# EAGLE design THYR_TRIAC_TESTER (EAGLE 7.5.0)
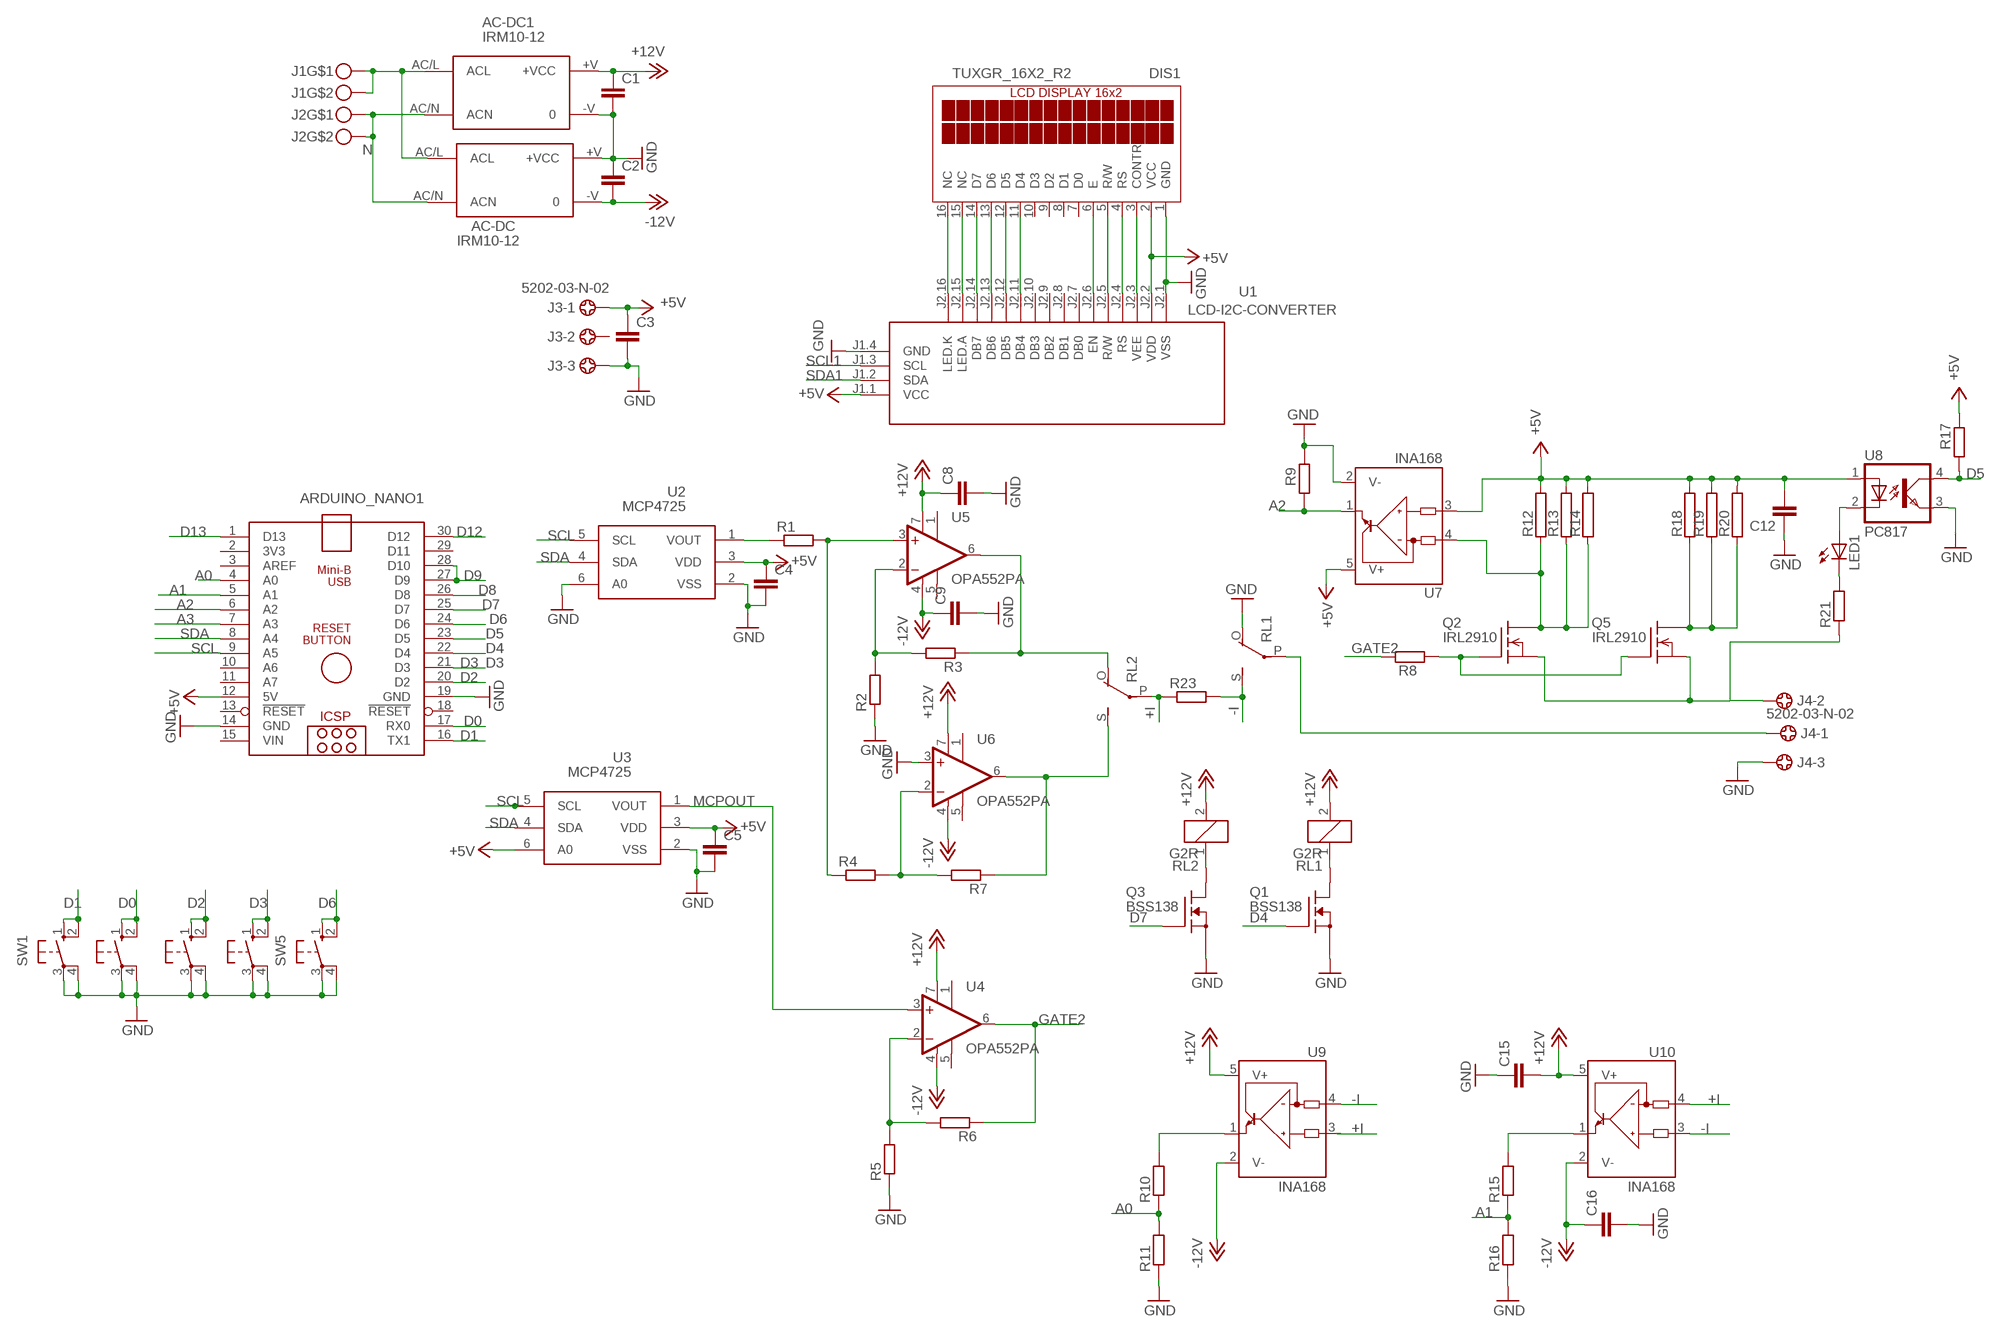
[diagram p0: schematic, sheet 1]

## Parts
AC-DC  IRM10-12  [IRM10-12]
AC-DC1  IRM10-12  [IRM10-12]
ARDUINO_NANO1  ARDUINO_NANO  [ARDUINO_NANO]
C1  C-EUC1206  [C1206]
C2  C-EUC1206  [C1206]
C3  C-EUC1206  [C1206]
C4  C-EUC1206  [C1206]
C5  C-EUC1206  [C1206]
C8  C-EUC1206  [C1206]
C9  C-EUC1206  [C1206]
C12  C-EUC1206  [C1206]
C15  C-EUC1206  [C1206]
C16  C-EUC1206  [C1206]
DIS1  TUXGR_16X2_R2  [TUXGR_16X2_R2]
J1  MKDSN1,5-2-5,08  [MKDSN1,5-2-5,08]
J2  MKDSN1,5-2-5,08  [MKDSN1,5-2-5,08]
J3  5202-03-N-02  [5202-03-N-02]
J4  5202-03-N-02  [5202-03-N-02]
LED1  LED5MM  [LED5MM]
Q1  BSS138  [SOT23]
Q2  IRL2910  SUP75N06-08  [TO220]
Q3  BSS138  [SOT23]
Q5  IRL2910  SUP75N06-08  [TO220]
R1  R-EU_M1206  [M1206]
R2  R-EU_M1206  [M1206]
R3  R-EU_M1206  [M1206]
R4  R-EU_M1206  [M1206]
R5  R-EU_M1206  [M1206]
R6  R-EU_M1206  [M1206]
R7  R-EU_M1206  [M1206]
R8  R-EU_M1206  [M1206]
R9  R-EU_M1206  [M1206]
R10  R-EU_M1206  [M1206]
R11  R-EU_M1206  [M1206]
R12  RRWM10X65  [RWM10X65]
R13  RRWM10X65  [RWM10X65]
R14  RRWM10X65  [RWM10X65]
R15  R-EU_M1206  [M1206]
R16  R-EU_M1206  [M1206]
R17  R-EU_M1206  [M1206]
R18  RRWM10X65  [RWM10X65]
R19  RRWM10X65  [RWM10X65]
R20  RRWM10X65  [RWM10X65]
R21  R-EU_M1206  [M1206]
R23  R-EU_R2512  [R2512]
RL1  G2R  [G2R]
RL2  G2R  [G2R]
SW1  40-XX  [B3F-40XX]
SW2  40-XX  [B3F-40XX]
SW3  40-XX  [B3F-40XX]
SW4  40-XX  [B3F-40XX]
SW5  40-XX  [B3F-40XX]
U1  LCD-I2C-CONVERTER  [LCD-I2C-CONVERTER]
U2  MCP4725  [SOT23-6]
U3  MCP4725  [SOT23-6]
U4  OPA552PA  OPA627U  [SO08]
U5  OPA552PA  OPA627U  [SO08]
U6  OPA552PA  OPA627U  [SO08]
U7  INA168  [SOT23-5]
U8  PC817  [DIL04]
U9  INA168  [SOT23-5]
U10  INA168  [SOT23-5]

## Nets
+5V: ARDUINO_NANO1.12(5V) C3.1 C4.1 C5.1 C12.2 DIS1.2(VCC) J3.1 R12.2 R13.2 R14.2 R17.2 R18.2 R19.2 R20.2 U1.J1.1(VCC) U1.J2.2(VDD) U2.3(VDD) U3.3(VDD) U3.6(A0) U7.3(IN+) U7.5(V+) U8.1(A)
+12V: AC-DC1.+V(+VCC) C1.1 C8.1 C15.2 RL1.2 RL2.2 U4.7(V+) U5.7(V+) U6.7(V+) U9.5(V+) U10.5(V+)
+I: R23.1 RL2.P(2:P) U10.4(IN-)
-12V: AC-DC.-V C2.2 C9.1 C16.1 U4.4(V-) U5.4(V-) U6.4(V-) U9.2(V-) U10.2(V-)
-I: R23.2 RL1.S(2:S) U9.4(IN-) U10.3(IN+)
A0: ARDUINO_NANO1.4(A0) R10.1 R11.2
A1: ARDUINO_NANO1.5(A1) R15.1 R16.2
A2: ARDUINO_NANO1.6(A2) R9.1 U7.1(OUT)
A3: ARDUINO_NANO1.7(A3)
D0: ARDUINO_NANO1.17(RX0) SW2.1(S) SW2.2(S1)
D1: ARDUINO_NANO1.16(TX1) SW1.1(S) SW1.2(S1)
D2: ARDUINO_NANO1.20(D2) SW3.1(S) SW3.2(S1)
D3: ARDUINO_NANO1.21(D3) SW4.1(S) SW4.2(S1)
D4: ARDUINO_NANO1.22(D4) Q1.3(G)
D5: ARDUINO_NANO1.23(D5) R17.1 U8.4(COL)
D6: ARDUINO_NANO1.24(D6) SW5.1(S) SW5.2(S1)
D7: ARDUINO_NANO1.25(D7) Q3.3(G)
D8: ARDUINO_NANO1.26(D8)
D9: ARDUINO_NANO1.27(D9) ARDUINO_NANO1.28(D10)
D12: ARDUINO_NANO1.30(D12)
D13: ARDUINO_NANO1.1(D13)
GATE2: R6.1 R8.2 U4.6(OUT)
GND: AC-DC1.-V AC-DC.+V(+VCC) ARDUINO_NANO1.14(GND) ARDUINO_NANO1.19(GND) C1.2 C2.1 C3.2 C4.2 C5.2 C8.2 C9.2 C12.1 C15.1 C16.2 DIS1.1(GND) J3.3 J4.3 Q1.1(S) Q3.1(S) R2.1 R5.1 R9.2 R11.1 R16.1 RL1.O(2:O) SW1.3(P) SW1.4(P1) SW2.3(P) SW2.4(P1) SW3.3(P) SW3.4(P1) SW4.3(P) SW4.4(P1) SW5.3(P) SW5.4(P1) U1.J1.4(GND) U1.J2.1(VSS) U2.2(VSS) U2.6(A0) U3.2(VSS) U6.3(+IN) U7.2(V-) U8.3(EMIT)
MCPOUT: U3.1(VOUT) U4.3(+IN)
N: AC-DC1.AC/N(ACN) AC-DC.AC/N(ACN) J2.1 J2.2
N$1: R1.1 U2.1(VOUT)
N$2: R1.2 R4.1 U5.3(+IN)
N$3: R3.1 RL2.O(2:O) U5.6(OUT)
N$4: AC-DC1.AC/L(ACL) AC-DC.AC/L(ACL) J1.1 J1.2
N$5: R2.2 R3.2 U5.2(-IN)
N$6: Q3.2(D) RL2.1
N$7: R7.1 RL2.S(2:S) U6.6(OUT)
N$8: R4.2 R7.2 U6.2(-IN)
N$9: Q2.1(G) Q5.1(G) R8.1
N$10: R5.2 R6.2 U4.2(-IN)
N$11: R10.2 U9.1(OUT)
N$12: Q1.2(D) RL1.1
N$13: LED1.A U8.2(C)
N$14: Q2.2(D) R12.1 R13.1 R14.1 U7.4(IN-)
N$15: Q5.2(D) R18.1 R19.1 R20.1
N$16: LED1.K(C) R21.2
N$18: R15.2 U10.1(OUT)
N$19: J4.1 RL1.P(2:P)
N$20: J4.2 Q2.3(S) Q5.3(S) R21.1
N$31: DIS1.3(CONTR) U1.J2.3(VEE)
N$32: DIS1.4(RS) U1.J2.4(RS)
N$33: DIS1.5(R/W) U1.J2.5(R/W)
N$34: DIS1.6(E) U1.J2.6(EN)
N$35: DIS1.14(D7) U1.J2.14(DB7)
N$36: DIS1.13(D6) U1.J2.13(DB6)
N$37: DIS1.12(D5) U1.J2.12(DB5)
N$38: DIS1.11(D4) U1.J2.11(DB4)
N$39: DIS1.16(NC) U1.J2.16(LED.K)
N$40: DIS1.15(NC) U1.J2.15(LED.A)
SCL: ARDUINO_NANO1.9(A5) U2.5(SCL) U3.5(SCL)
SCL1: U1.J1.3(SCL)
SDA: ARDUINO_NANO1.8(A4) U2.4(SDA) U3.4(SDA)
SDA1: U1.J1.2(SDA)
Unconnected: ARDUINO_NANO1.2(3V3) ARDUINO_NANO1.3(AREF) ARDUINO_NANO1.10(A6) ARDUINO_NANO1.11(A7) ARDUINO_NANO1.13(!RESET) ARDUINO_NANO1.18(!RESET) ARDUINO_NANO1.29(D11) DIS1.7(D0) DIS1.8(D1) DIS1.9(D2) DIS1.10(D3) J3.2 U1.J2.7(DB0) U1.J2.8(DB1) U1.J2.9(DB2) U1.J2.10(DB3) U4.1(TRIM1) U4.5(TRIM2) U5.1(TRIM1) U5.5(TRIM2) U6.1(TRIM1) U6.5(TRIM2) U9.3(IN+)

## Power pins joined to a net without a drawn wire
VIN: ARDUINO_NANO1.15(VIN)

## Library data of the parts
AC-DC AC-DC1 = acdc:IRM10-12
ARDUINO_NANO1 = ArduinoNanoV30:ARDUINO_NANO: Arduino Nano V3.0 Overview: The Arduino Nano is a small, complete, and breadboard-friendly board based on the ATmega328 (Arduino Nano 3.x) or ATmega168 (Arduino Nano 2.x). It has more or less the same functionality of the Arduino Duemilanove, but in a different package. It lacks only a DC power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
C1-C5 C8 C9 C12 C15 C16 = rcl:C-EU: CAPACITOR, European symbol
DIS1 = display-lcd:TUXGR_16X2_R2: Tuxgraphics LCD display 16x2 characters reflective, without background light Source: tuxgr_12x2_r2.pdf; OC_FARNELL: unknown; OC_NEWARK: unknown
J1 J2 = con-phoenix-508:MKDSN1,5-2-5,08
J3 J4 = con-ebyelectro:5202-03-N-02: Barrier Blocks Sreies 5202 Source: http://www.ebyelectro.com/PDF/5202-XX-N-02.pdf; OC_FARNELL: unknown; OC_NEWARK: unknown
LED1 = led:LED: LED
Q1 Q3 = transistor-fet:BSS138
Q2 Q5 = transistor-fet:SUP75N06-08: N-Channel Enhancement MOSFET 60V; 75A; 0,008Ohm
R1-R11 R15-R17 R21 R23 = rcl:R-EU_: RESISTOR, European symbol
R12-R14 R18-R20 = resistor-power:R: Power Resitor; OC_FARNELL: unknown; OC_NEWARK: unknown
RL1 RL2 = relay:G2R: RELAY 1 x switch, Omron; OC_FARNELL: 1569185; OC_NEWARK: unknown
SW1-SW5 = switch-omron:40-XX: OMRON SWITCH; MF: OMRON COMPONENTS USA; MPN: B3F-4000; OC_FARNELL: 176434; OC_NEWARK: 36K3105
U1 = diy-modules:LCD-I2C-CONVERTER: I2C Bus to 4-Bit Parallel LCD Interface with LED backlight driver
U2 U3 = linear:MCP4725
U4-U6 = burr-brown:OPA627: Difet(R) Operational Amplifiers Precision, High-Speed; MF: TEXAS INSTRUMENTS; MPN: OPA627AU; OC_FARNELL: 1207067; OC_NEWARK: 30C4516
U7 U9 U10 = burr-brown:INA168: High-Side Measurement Current Shunt Monitor; MF: TEXAS INSTRUMENTS; MPN: INA168NA/250; OC_FARNELL: 4375737; OC_NEWARK: 35C1744
U8 = optocoupler:PC817: SHARP OPTO COUPLER; MPN: PC817X4J000F; OC_FARNELL: 9707727; OC_NEWARK: 97K7059

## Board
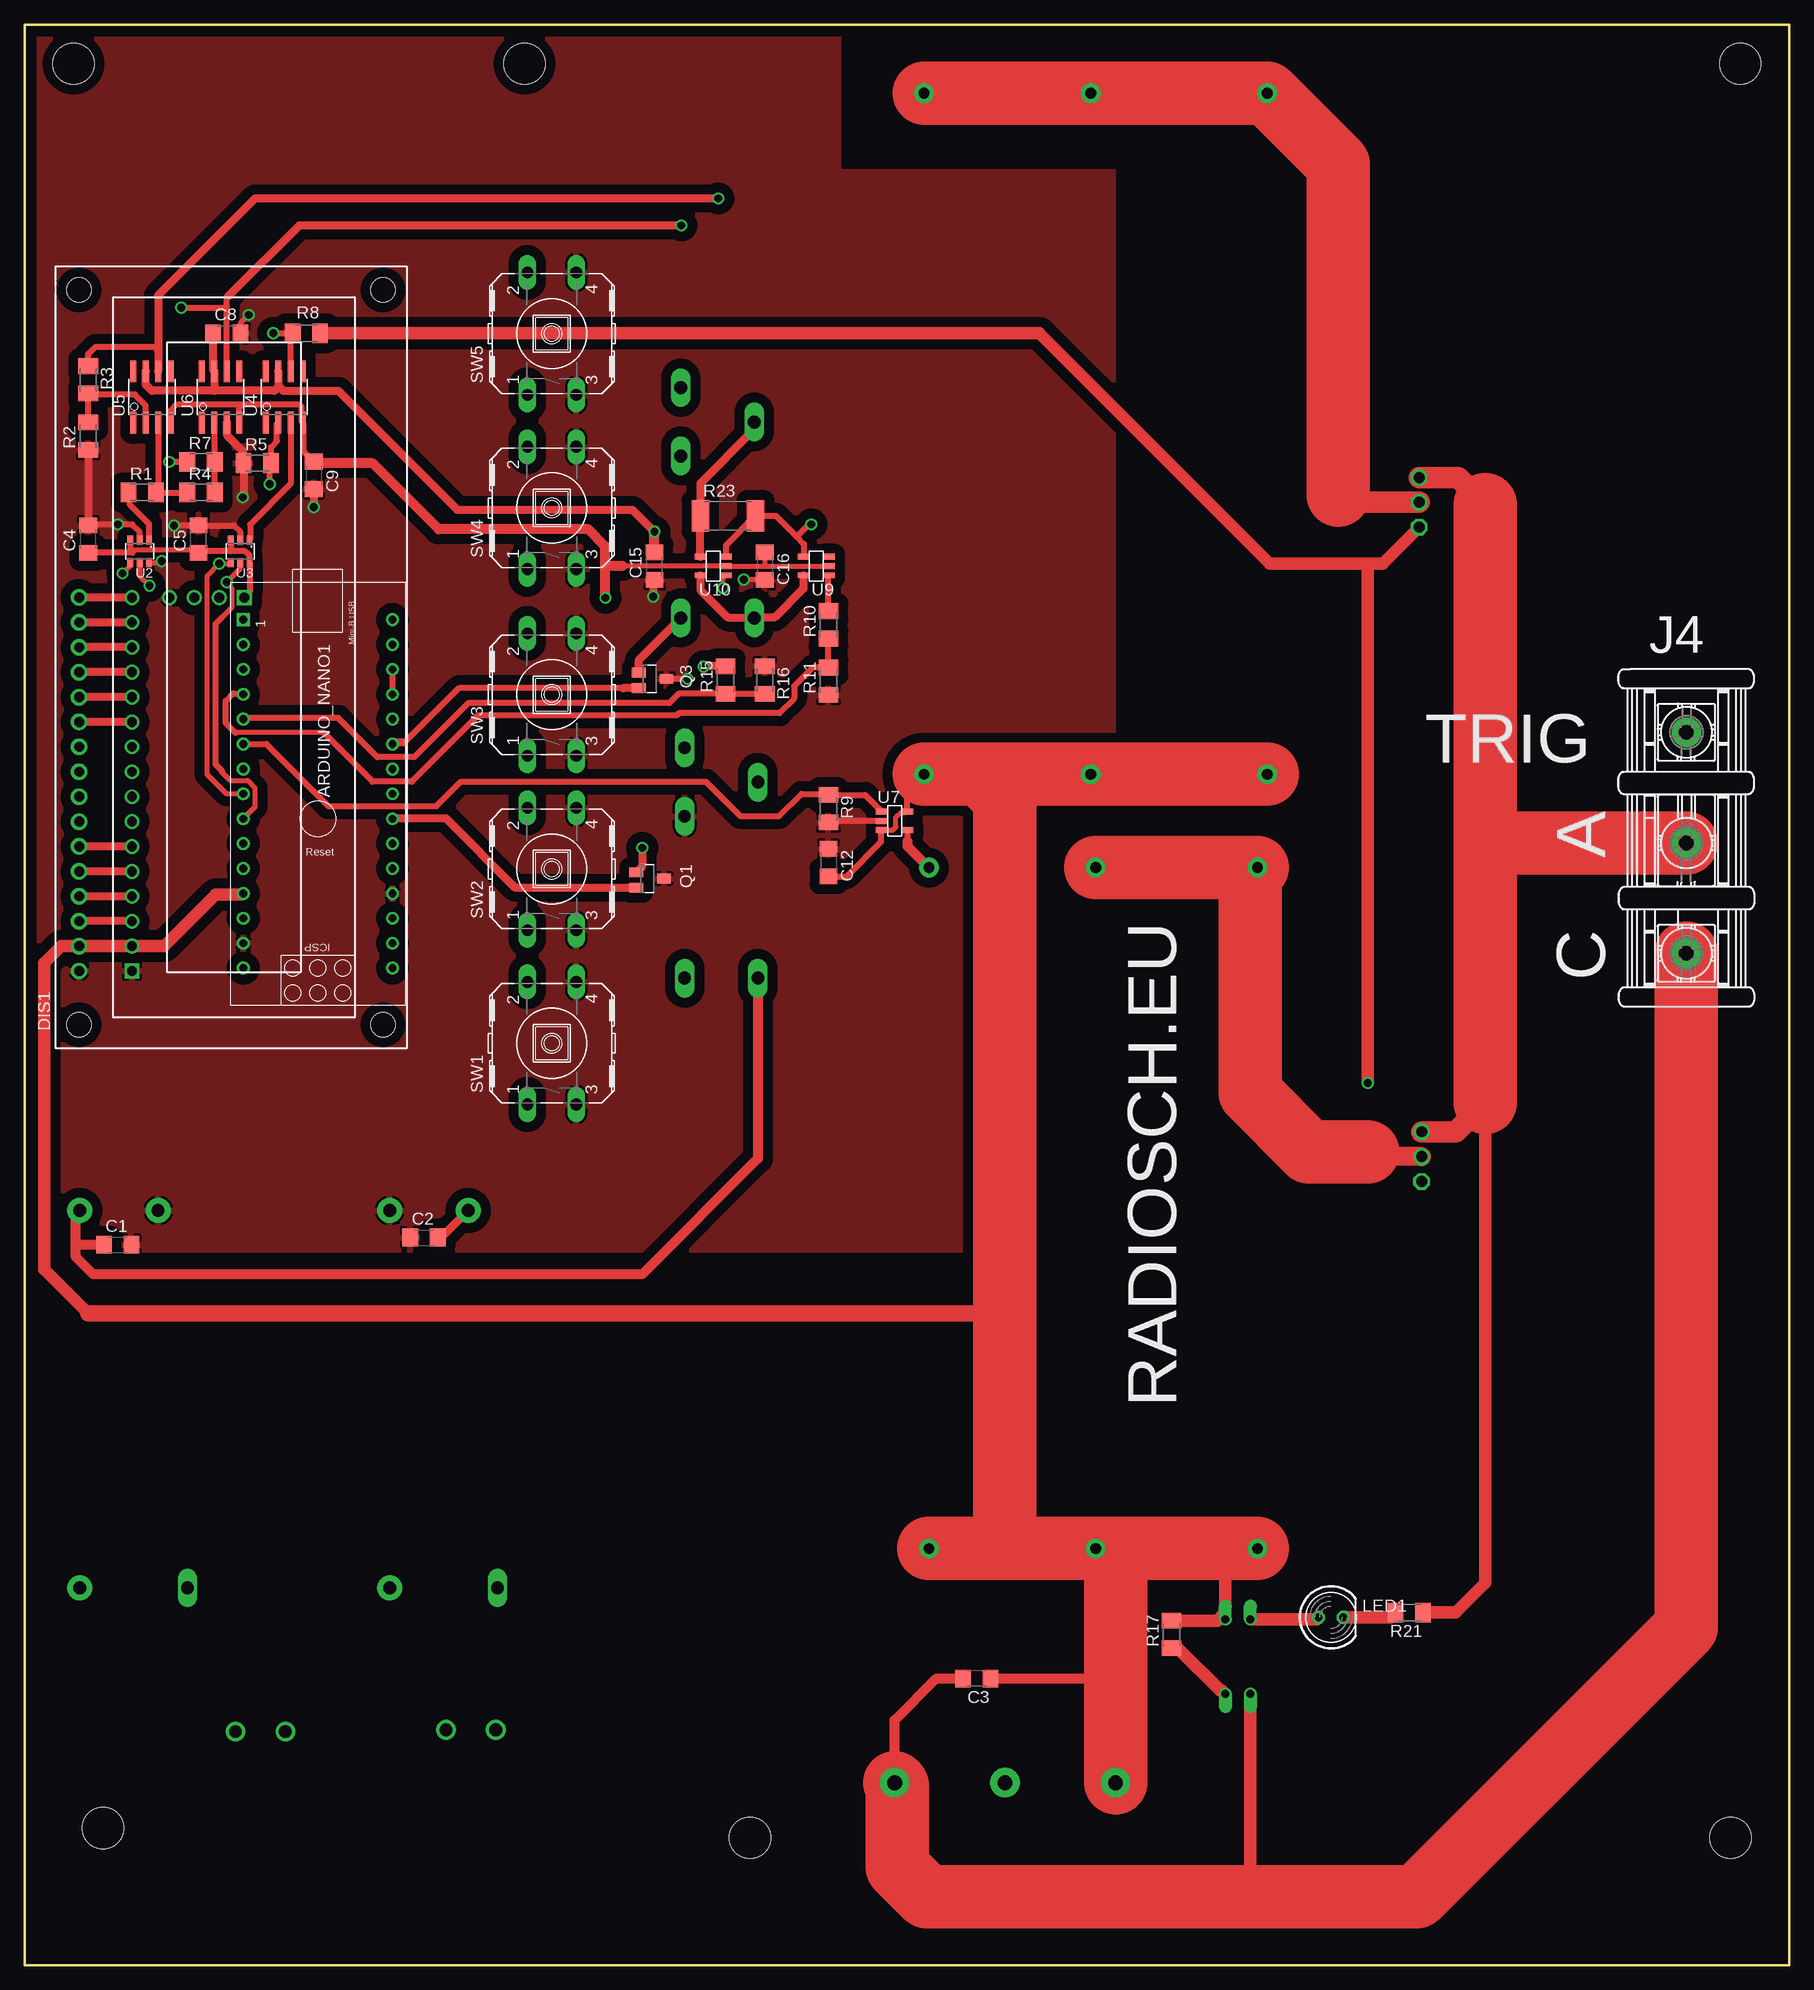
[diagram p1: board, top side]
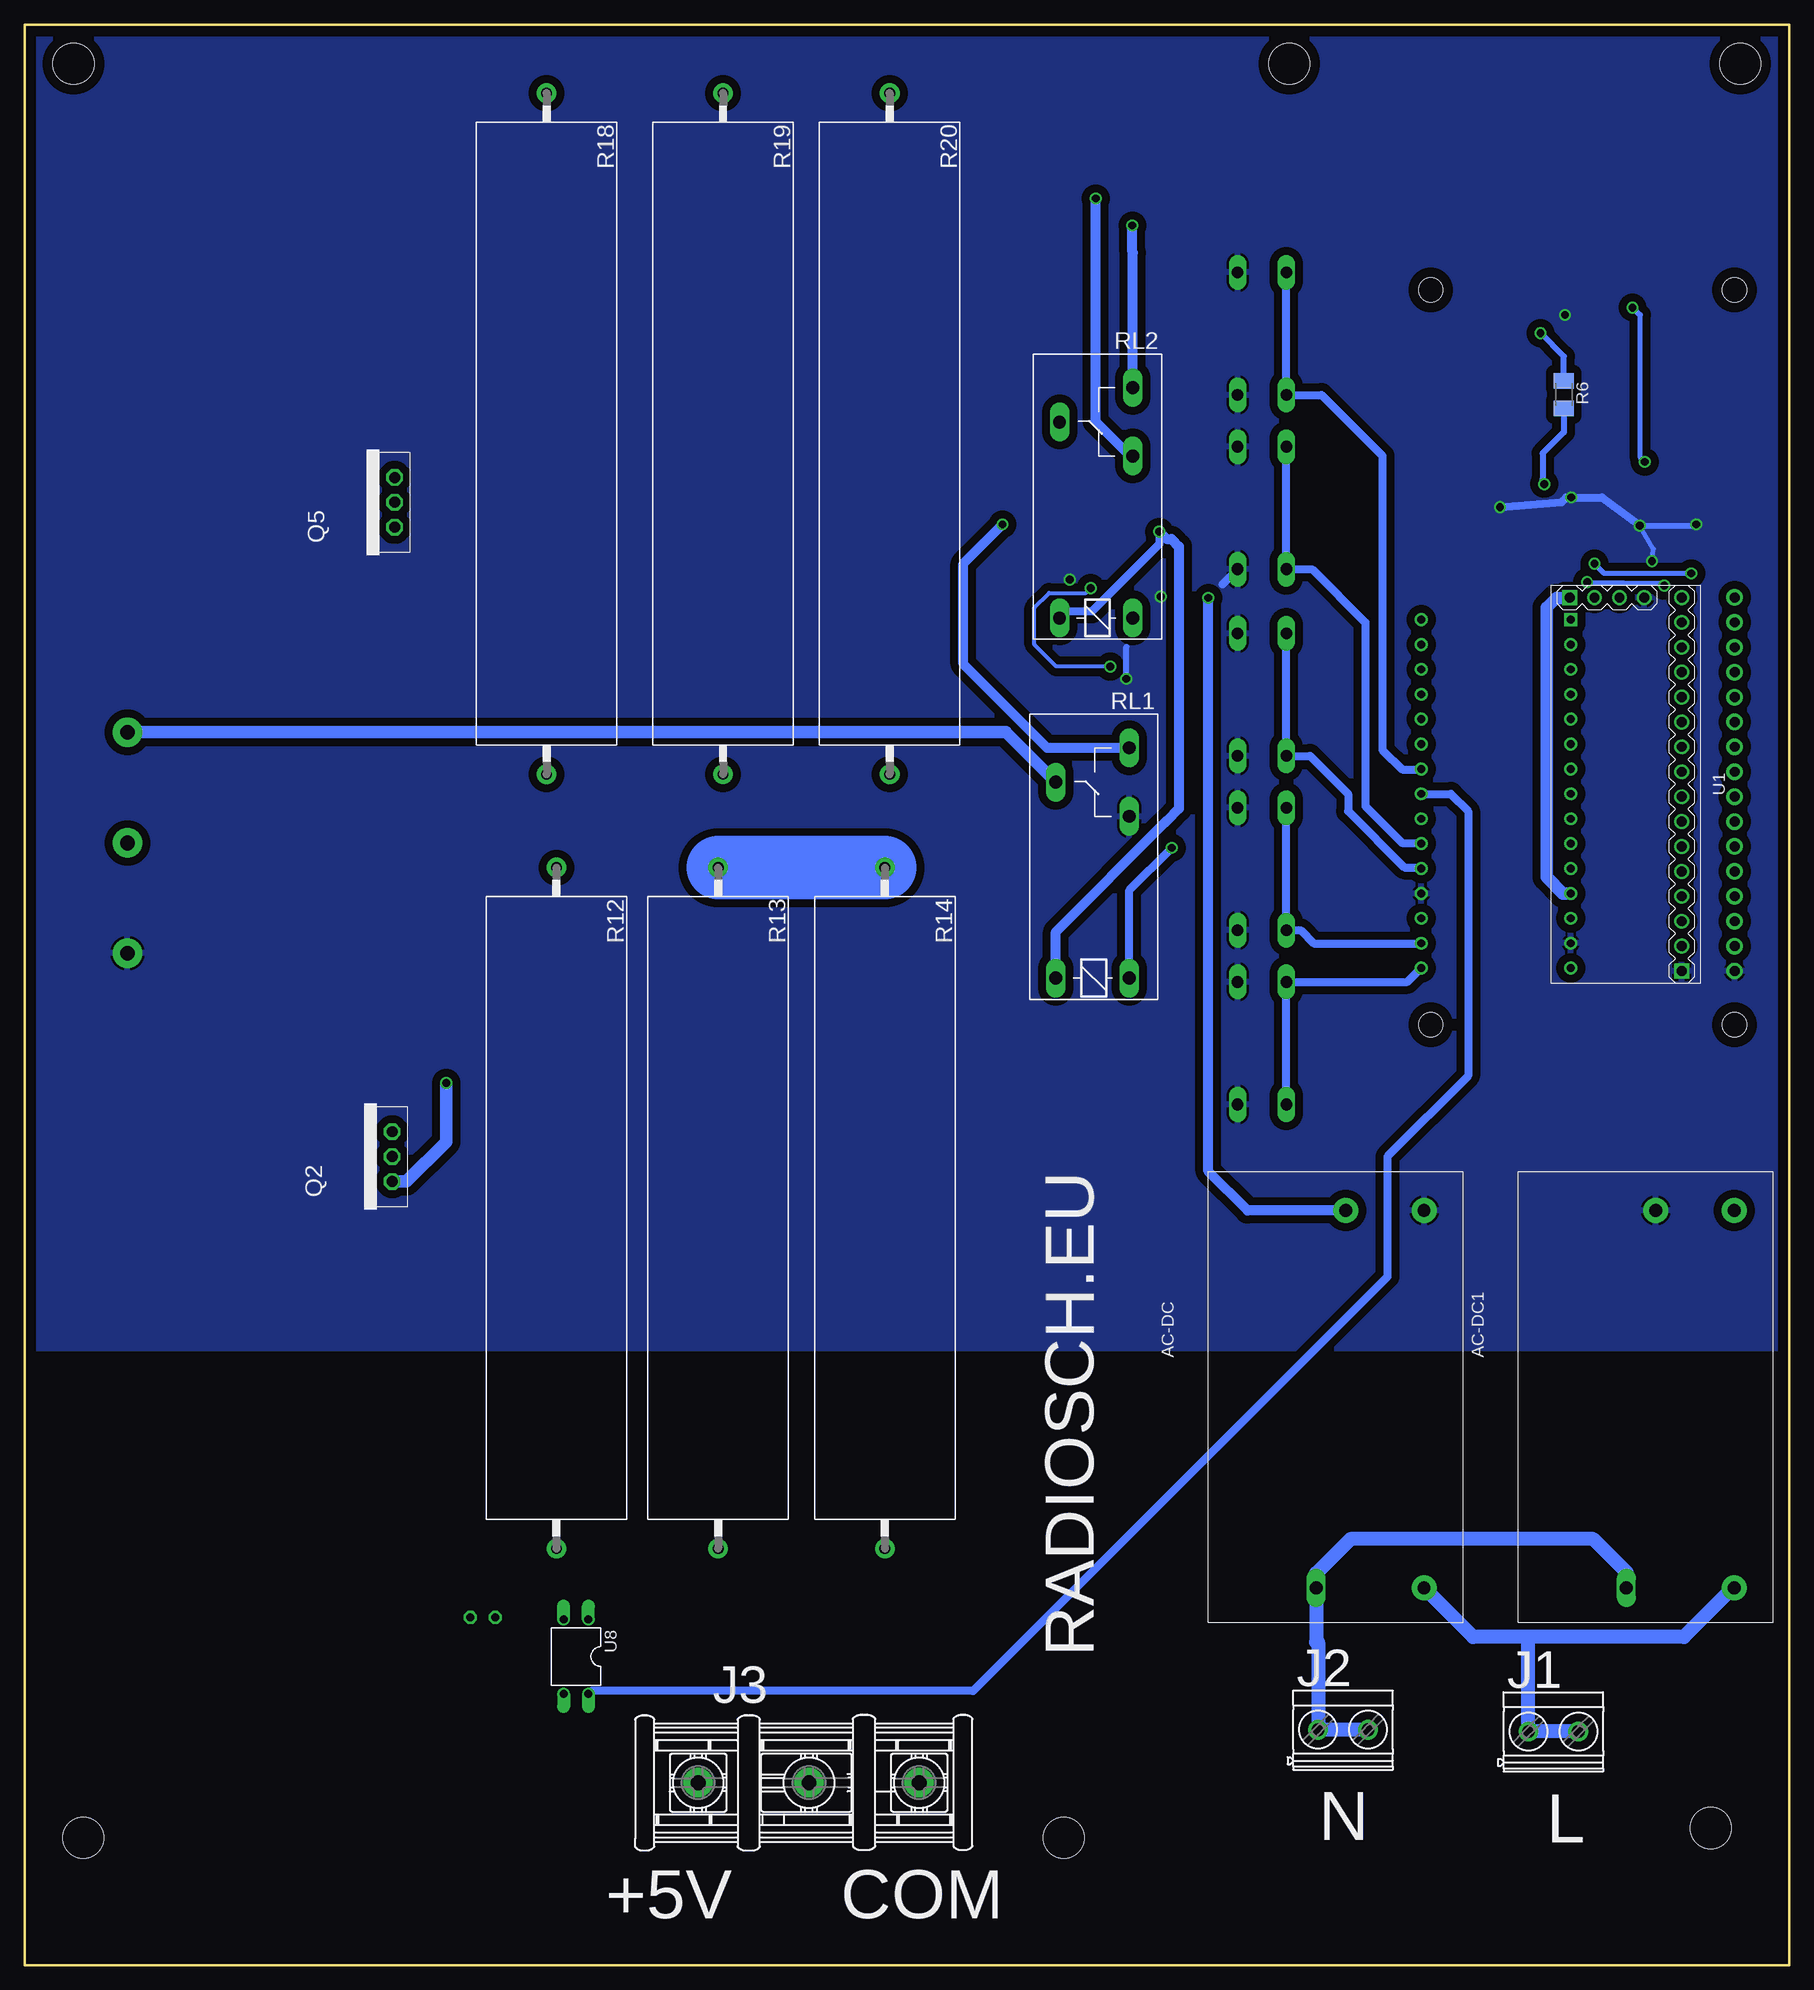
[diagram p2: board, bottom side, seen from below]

Size 180 x 198 mm. Coordinates in mm from the lower left corner, seen from the top.
Outline: 0,0 180,0 180,198 0,198 0,0
Copper layers (1*16): Top 0.035mm / dielectric 1.5mm / Bottom 0.035mm
Design rules "default": minimum track width 10mil, minimum drill 24mil, track to track 8mil, track to pad 8mil, pad to pad 8mil, via to via 8mil, smd to smd 8mil, copper to edge 40mil, drill to drill 8mil, minimum pad ring 10mil, minimum via ring 8mil, stop-mask expansion 4mil, vias tented up to drill 0mil, thermal gap 10mil
Holes 4.2 mm at 5,194 51,194 175,194 8,14 74,13 174,13

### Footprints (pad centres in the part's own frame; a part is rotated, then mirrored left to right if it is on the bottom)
IRM10-12 = drill 1.3 pad 2.54: +V 38.5,0; -V 38.5,8; AC/L 0,0 | drill 1.3 long: AC/N 0,11
ARDUINO_NANO = drill 0.8 square: 1 -20.32,-7.62 | drill 0.8: 2 -17.78,-7.62; 3 -15.24,-7.62; 4 -12.7,-7.62; 5 -10.16,-7.62; 6 -7.62,-7.62; 7 -5.08,-7.62; 8 -2.54,-7.62; 9 0,-7.62; 10 2.54,-7.62; 11 5.08,-7.62; 12 7.62,-7.62; 13 10.16,-7.62; 14 12.7,-7.62; 15 15.24,-7.62; 16 15.24,7.62; 17 12.7,7.62; 18 10.16,7.62; 19 7.62,7.62; 20 5.08,7.62; 21 2.54,7.62; 22 0,7.62; 23 -2.54,7.62; 24 -5.08,7.62; 25 -7.62,7.62; 26 -10.16,7.62; 27 -12.7,7.62; 28 -15.24,7.62; 29 -17.78,7.62; 30 -20.32,7.62
C1206 = smd 1.6 x 1.8: 1 -1.4,0; 2 1.4,0
TUXGR_16X2_R2 = drill 1 pad 1.676: 1 -32,15.5; 2 -29.46,15.5; 3 -26.92,15.5; 4 -24.38,15.5; 5 -21.84,15.5; 6 -19.3,15.5; 7 -16.76,15.5; 8 -14.22,15.5; 9 -11.68,15.5; 10 -9.14,15.5; 11 -6.6,15.5; 12 -4.06,15.5; 13 -1.52,15.5; 14 1.02,15.5; 15 3.56,15.5; 16 6.1,15.5 | hole 2.5: -37.5,-15.5; 37.5,-15.5; -37.5,15.5; 37.5,15.5
MKDSN1,5-2-5,08 = drill 1.3 pad 2: 1 -2.561,0.025; 2 2.519,0.025
5202-03-N-02 = drill 1.5 pad 3: 1 -9.29,0; 2 2,0; 3 13.25,0
LED5MM = drill 0.813 octagon: A -1.27,0; K 1.27,0
SOT23 = smd 1 x 1.4: 1 0,1.735; 2 -0.632,-1.1; 3 0.95,-1.1
TO220 = drill 1.118 octagon: 1 -2.54,0; 2 0,0; 3 2.54,0
M1206 = smd 1.6 x 2: 1 -1.4,0; 2 1.4,0
RWM10X65 = drill 1.1 pad 2: 1 -34.74,0; 2 34.74,0
R2512 = smd 1.8 x 3.2: 1 -2.8,0; 2 2.8,0
G2R = drill 1.321 long: 1 -2.54,-3.683; 2 -2.54,3.81; O 13.97,-3.683; P 17.45,3.81; S 20.955,-3.683
B3F-40XX = drill 1.194 long: 1 -6.248,2.489; 2 6.248,2.489; 3 -6.248,-2.489; 4 6.248,-2.489
LCD-I2C-CONVERTER = drill 1 square: J1.1 -19.05,-5.08; J2.1 19.05,6.35 | drill 1: J1.2 -19.05,-2.54; J1.3 -19.05,0; J1.4 -19.05,2.54; J2.2 16.51,6.35; J2.3 13.97,6.35; J2.4 11.43,6.35; J2.5 8.89,6.35; J2.6 6.35,6.35; J2.7 3.81,6.35; J2.8 1.27,6.35; J2.9 -1.27,6.35; J2.10 -3.81,6.35; J2.11 -6.35,6.35; J2.12 -8.89,6.35; J2.13 -11.43,6.35; J2.14 -13.97,6.35; J2.15 -16.51,6.35; J2.16 -19.05,6.35
SOT23-6 = smd 0.6 x 0.9: 1 -0.95,-1.15; 2 0,-1.15; 3 0.95,-1.15; 4 0.95,1.15; 5 0,1.15; 6 -0.95,1.15
SO08 = smd 0.61 x 2.21: 1 -1.905,-2.616; 2 -0.635,-2.616; 3 0.635,-2.616; 4 1.905,-2.616; 5 1.905,2.616; 6 0.635,2.616; 7 -0.635,2.616; 8 -1.905,2.616
SOT23-5 = smd 0.6 x 1.2: 1 -0.95,-1.306; 2 0,-1.306; 3 0.95,-1.306; 4 0.95,1.306; 5 -0.95,1.306
DIL04 = drill 0.813 offset: 1 -1.27,-3.81; 2 1.27,-3.81; 3 1.27,3.81; 4 -1.27,3.81

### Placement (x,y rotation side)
AC-DC  37.25,38.5 90 bottom
AC-DC1  5.62,38.5 90 bottom
ARDUINO_NANO1  29.92,116.97 270 top
C1  9.5,73.5 0 top
C2  40.75,74.25 0 top
C3  97.12,29.25 180 top
C4  6.5,145.5 90 top
C5  17.75,145.5 90 top
C8  20.62,166.5 0 top
C9  29.5,152 270 top
C12  82,112.5 270 top
C15  64.25,142.75 90 top
C16  75.5,142.75 270 top
DIS1  21.07,133.44 90 top
J1  24.04,23.82 0 bottom
J2  45.5,24 0 bottom
J3  102,18.62 0 bottom
J4  169.5,116.5 270 top
LED1  133.25,35.5 0 top
Q1  63.5,110.88 270 top
Q2  142.5,82.5 90 bottom
Q3  63.75,131.25 270 top
Q5  142.25,149.25 90 bottom
R1  12,150.25 0 top
R2  6.5,156 90 top
R3  6.5,161.75 270 top
R4  18,150.25 0 top
R5  23.75,153.25 0 top
R6  23,160.25 270 bottom
R7  18,153.38 0 top
R8  28.75,166.5 180 top
R9  82,118 270 top
R10  82,136.75 90 top
R11  82,131 90 top
R12  125.75,77.25 270 bottom
R13  109.25,77.25 270 bottom
R14  92.25,77.25 270 bottom
R15  71.5,131.12 90 top
R16  75.5,131.12 270 top
R17  117,33.75 90 top
R18  126.75,156.25 270 bottom
R19  108.75,156.25 270 bottom
R20  91.75,156.25 270 bottom
R21  141.25,36 180 top
R23  71.75,147.88 0 top
RL1  71,103.25 90 bottom
RL2  70.62,140 90 bottom
SW1  53.78,94.07 90 top
SW2  53.78,111.85 90 top
SW3  53.78,129.63 90 top
SW4  53.78,148.68 90 top
SW5  53.78,166.46 90 top
U1  17.32,120.49 270 bottom
U2  11.75,144.25 180 top
U3  22,144.25 180 top
U4  26.5,160 0 top
U5  13,160 0 top
U6  20,160 0 top
U7  88.75,116.75 270 top
U8  123.75,31.5 180 bottom
U9  80.75,142.75 90 top
U10  70.25,142.75 90 top

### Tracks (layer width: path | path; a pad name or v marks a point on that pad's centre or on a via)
+5V
  Top 0.5: C5.1 17.27,144.1 17,144.38 11.28,144.38 11,144.1 10.8,144.3 | U7.3 88.55,115.8 88.88,116.12 88.88,117.12 89.38,117.62 89.98,117.62 U7.5
  Top 0.61: U7.5 90.06,119.32 92.25,121.51 | C12.2 83.85,111.1 87.38,114.62 87.38,115.73 U7.3 | U1.J1.1 22.95,140.09 U3.6 22.95,143.8 22.5,144.25 21,144.25 | 21,144.25 18.4,144.25 C5.1 | U3.3 21.05,144.3 21,144.25 | 11,144.1 C4.1 | U2.3 10.8,144.3
  Top 1.016: C3.1 111.04,29.25 111.29,29
  Top 1.27: U8.1 122.48,36 | 122.48,36 122.48,42.03 122,42.51 | R17.2 121.63,35.15 122.48,36 | 6.5,66.5 2,71 2,102.25 3.73,103.98 DIS1.2 U1.J2.2 14.23,103.98 19.5,109.25 22.2,109.25 ARDUINO_NANO1.12
  Top 1.676: 6.5,66.5 98.25,66.5 98.5,66.25 100,66.25
  Top 6.452: R20.2 92.25,121.51 99,121.51 | 99,121.51 R19.2 R18.2 | R12.2 122,42.51 110,42.51 | 110,42.51 R13.2 R14.2 99.51,42.51 100,43 100,66.25 100,119 98,121 99,121 99,121.51 | J3.1 111.29,29 111.29,41.22 110,42.51
  Bottom 1.27: ARDUINO_NANO1.12 23.1,109.35 24.75,111 24.75,138.5 23.75,139.5 22.44,139.5 U1.J1.1
+12V  (via drill 0.8)
  Top 0.813: 19.38,160.62 19.36,160.63 U6.7 19.23,162.76 C8.1 | 19.38,160.62 13,160.62 12.38,161.25 12.38,162.61 U5.7 | U4.7 25.86,160.99 | 25.86,160.99 25.5,160.62 19.38,160.62 | 25.86,160.99 26.01,160.99 26.38,160.62 32,160.62 44.12,148.5 62,148.5 v64.25,146.25 | U10.5 68.94,140.31 71.75,137.5 74.39,137.5 RL2.2 74.47,137.5 76.5,137.5 79.44,140.44 U9.5
  Top 1.016: RL1.2 74.81,82.31 63,70.5 7,70.5 5.25,72.25 5.25,73.5 | 5.25,73.5 5.25,76.62 AC-DC1.+V | C1.1 5.25,73.5 | C15.2 v64.25,146.25
  Bottom 0.813: v64.25,146.25 64.25,145 71.12,138.12 73.77,138.12 RL2.2
  Bottom 1.016: RL1.2 74.81,105.44 63.62,116.62 63.5,116.75 62.25,118 62.25,144.75 63,145.5 63.5,145.5 v64.25,146.25
+I
  Top 0.813: U10.4 R23.1 68.95,151.2 74.25,156.5 74.25,157.26 RL2.P
-12V  (via drill 0.8)
  Top 0.5: 61,142.75 U10.2 75.38,142.75 | 29.65,153.25 32.75,153.25 | 75.38,142.75 U9.2 | C16.1 75.5,142.88 75.38,142.75
  Top 0.61: U5.4 14.9,158.66 15.5,159.25 22.25,159.25 | 22.25,159.25 28,159.25 28.25,159 28.25,157.54 U4.4 28.41,154.5 C9.1 | U6.4 21.91,158.91 22.25,159.25
  Top 0.813: C2.2 42.5,74.25 AC-DC.-V
  Top 1.016: v59.25,139.5 59.25,142.75 | 59.25,142.75 59.25,144.75 57.5,146.5 42.25,146.5 35.5,153.25 29.65,153.25 C9.1 | 61,142.75 59.25,142.75
  Bottom 1.016: AC-DC.-V 55.25,77 59.25,81 v59.25,139.5
-I  (via drill 0.8)
  Top 0.61: U10.3 71.56,144.88 R23.2 76.62,147.88 78.75,145.75 | 78.75,145.75 79.5,145 79.5,143.76 U9.4 | v80.25,147 80,147 78.75,145.75
  Bottom 1.016: RL1.S 75.7,124.2 84.25,132.75 84.25,143 v80.25,147
A0
  Top 0.5: 30.5,125.75 21.5,125.75
  Top 0.61: R10.1 R11.2 80.4,132.4 78.5,130.5 78.5,129.25 77,127.75 66.75,127.75 66.5,127.5 46.25,127.5 39.5,120.75 35.5,120.75 30.5,125.75 | 21.5,125.75 20.5,126.75 20.5,129 21.25,129.75 22.22,129.75 ARDUINO_NANO1.4
A1
  Top 0.61: ARDUINO_NANO1.5 22.42,127.25 32,127.25 36,123.25 39.75,123.25 45.25,128.75 65.75,128.75 66.72,129.72 R15.1 R16.2
A2
  Top 0.61: U7.1 85.74,119.4 R9.1 81.9,119.5 79.25,119.5 77,117.25 73,117.25 69.5,120.75 44.5,120.75 42,118.25 31,118.25 24.66,124.59 ARDUINO_NANO1.6
D0
  Bottom 0.813: ARDUINO_NANO1.17 37.56,104.25 48.5,104.25 49.85,105.6 SW2.1 SW2.2
D1
  Bottom 0.813: ARDUINO_NANO1.16 38.95,100.32 SW1.2 SW1.1
D2
  Bottom 0.813: ARDUINO_NANO1.20 37.65,112 39.25,112 45,117.75 45,119.5 48.88,123.38 SW3.1 SW3.2
D3
  Bottom 0.813: ARDUINO_NANO1.21 37.61,114.5 39.5,114.5 43.25,118.25 43.25,137 48.68,142.43 SW4.1 SW4.2
D4
  Top 0.813: Q1.3 50.08,109.92 43,117 37.57,117 ARDUINO_NANO1.22
D5
  Top 1.27: R17.1 117.65,32.35 122,28 122.17,28 U8.4
  Bottom 0.813: ARDUINO_NANO1.23 34.51,119.51 32.75,117.75 32.75,90.75 41,82.5 41,70.25 83.25,28 122.17,28 U8.4
D6
  Bottom 0.813: ARDUINO_NANO1.24 37.59,122 39.5,122 41.5,124 41.5,154 47.71,160.21 SW5.1 SW5.2
D7
  Top 0.61: 61.05,130.3 44.3,130.3 38.75,124.75
  Top 0.813: Q3.3 61.05,130.3 | 38.75,124.75 37.7,124.75 ARDUINO_NANO1.25
D9
  Top 0.61: ARDUINO_NANO1.27 ARDUINO_NANO1.28
GATE2  (via drill 0.8)
  Top 0.61: U4.6 27.14,166.28 R8.2 v25.38,166.5
  Bottom 0.61: R6.1 23,164.12 v25.38,166.5
GND  (via drill 0.8)
  Top 0.5: U2.6 13.78,143.1 v14,143.25 | C8.2 22.02,167.53 v22.88,168.38 | C16.2 73.6,141.35 v73.38,141.38
  Top 0.61: U7.2 82.75,116.75 82.62,116.62 82.03,116.62 R9.2 | U2.2 11.75,146.25 11,147 v9.5,147 6.6,147 C4.2 | v15.25,146.88 16.27,146.9 C5.2 21.35,146.9 22,146.25 U3.2 | Q3.1 v67.62,131.25
  Top 0.813: U6.3 20.64,156.12 22.25,154.5 22.25,153.35 R5.1 22.35,149.85 v22.25,149.75 | C9.2 v29.5,148.75 | R2.1 C4.2 | C15.1 64.12,141.22 v64.12,139.62
  Top 1.016: J3.3 88.75,25 93,29.25 C3.2
  Top 1.27: U8.3 125.02,9.02 125,9 125,8 124,7
  Top 6.452: J3.3 89,18.38 89,10 92,7 124,7 142,7 169.5,34.5 J4.3
  Bottom 0.5: v14,143.25 13.88,144.5 v15.25,146.88
  Bottom 0.61: v15.25,146.88 9.62,146.88 v9.5,147 | v67.62,131.25 67.62,134.5
  Bottom 0.813: v15.25,146.88 19.12,149.75 v22.25,149.75 22.75,149.75 23.25,149.25 v29.5,148.75 | 57.83,140.88 SW4.3
  pour Bottom (isolate 0.813): 1,197 180,197 180,63 1,63
  pour Top (isolate 1.016): 1,197 83,197 83,183 111,183 111,73 1,73
MCPOUT
  Top 0.61: U4.3 27.14,151.13 23,147 23,145.45 U3.1
N
  Bottom 1.422: AC-DC1.AC/N 16.62,40.12 20,43.5 44.75,43.5 48.25,40 AC-DC.AC/N 48.25,32.96 48.06,32.96 J2.1 J2.2
N$1
  Top 0.61: U2.1 12.7,147.05 10.75,149 10.75,150.1 R1.1
N$2
  Top 0.61: U5.3 13.63,150.49 R1.2 R4.1
N$3  (via drill 0.8)
  Top 0.61: R3.1 6.5,164.38 7.25,165.12 13.25,165.12 13.62,164.75
  Top 0.813: v70.75,180.25 23.5,180.25 13.62,170.38 13.62,164.75 U5.6
  Bottom 1.016: RL2.O 67.22,153.97 70.75,157.5 v70.75,180.25
N$4
  Bottom 1.422: AC-DC1.AC/L 5.75,38.5 10.75,33.5 26.75,33.5 | 26.75,33.5 32.25,33.5 AC-DC.AC/L | 26.75,33.5 26.6,33.35 J1.1 J1.2
N$5
  Top 0.61: U5.2 12.37,159.13 11.25,160.25 6.6,160.25 R3.2 6.4,160.25 5.88,160.25 6.5,159.62 R2.2
N$6
  Top 0.813: Q3.2 62.65,133.17 RL2.1
N$7  (via drill 0.8)
  Top 0.61: U6.6 20.64,169.25 | 20.64,169.25 20.64,170.13 20.75,170.25 | R7.1 v14.75,153.38 | v16,169.12 20.51,169.12 20.64,169.25
  Top 0.813: v67,177.5 28,177.5 20.75,170.25
  Bottom 0.5: 15.25,168.38 15.25,153.88 v14.75,153.38
  Bottom 0.61: 15.25,168.38 v16,169.12
  Bottom 1.016: RL2.S 66.94,174.69 67,174.75 v67,177.5
N$8
  Top 0.61: U6.2 19.4,157.35 R7.2 R4.2
N$9  (via drill 0.8)
  Top 1.27: R8.1 103.5,166.5 127,143 137,143 | 137,143 138.54,143 Q5.1 | v137,90 137,143
  Bottom 1.27: Q2.1 141.04,79.96 137,84 v137,90
N$10  (via drill 0.8)
  Top 0.61: U4.2 25.75,157.27 25.75,155.5 25.15,154.9 R5.2 25,153.1 v25,151.12
  Bottom 0.61: R6.2 23,156.4 25.15,154.25 25.15,151.65 v25,151.12
N$11
  Top 0.61: R10.2 82,141.74 U9.1
N$12  (via drill 0.8)
  Top 0.813: v63,114 63,112.11 Q1.2
  Bottom 0.813: RL1.1 67.32,109.68 v63,114
N$13
  Top 1.27: U8.2 131.79,35.31 LED1.A
N$14
  Top 0.61: U7.4 90.06,114.68
  Top 1.016: 90.06,114.68 90.06,114.18 R14.1
  Top 1.93: Q2.2 137.5,82.5 137,83
  Top 6.452: R13.1 125,111.99 | 125,111.99 R12.1 | 137,83 131,83 125,89 125,111.99
  Bottom 6.452: R13.1 R14.1
N$15
  Top 2.184: Q5.2 134.75,149.25 134,150
  Top 6.452: R20.1 R19.1 | R19.1 108.99,190.99 109,191 | R19.1 R18.1 134,183.74 134,150
N$16
  Top 1.27: LED1.K 139.35,35.5 R21.2
N$18  (via drill 0.8)
  Top 0.406: v71.25,140.5 71.25,141.49 U10.1
  Top 0.813: R15.2 69.78,132.53 v69.25,132.5
  Bottom 0.406: v69.25,132.5 74.75,132.5 77,134.75 77,138.5 75.5,140 71.75,140 v71.25,140.5
N$19
  Bottom 1.27: J4.1 79.9,125.79 RL1.P
N$20
  Top 1.27: R21.1 146,36 149,39 149,89
  Top 2.184: Q5.3 146.21,151.79 149,149 | 149,88 146,85 142.54,85 Q2.3 | 149.79,125.79 149,125
  Top 6.452: 149,149 149,125 149,115 | 149,115 149,89 149,88 | J4.2 149.5,114.5 149,115
N$31
  Top 0.813: U1.J2.3 DIS1.3
N$32
  Top 0.813: U1.J2.4 DIS1.4
N$33
  Top 0.813: U1.J2.5 DIS1.5
N$34
  Top 0.813: U1.J2.6 DIS1.6
N$35
  Top 0.813: U1.J2.14 DIS1.14
N$36
  Top 0.813: U1.J2.13 DIS1.13
N$37
  Top 0.813: U1.J2.12 DIS1.12
N$38
  Top 0.813: U1.J2.11 DIS1.11
N$39
  Top 0.813: U1.J2.16 DIS1.16
N$40
  Top 0.813: U1.J2.15 DIS1.15
SCL  (via drill 0.8)
  Top 0.5: U3.5 22,142.5 v20.62,141.12 20.62,141 21.12,140.5 21.12,138.5 20.12,137.5 | 20.12,121.75 21,120.88 22.75,120.88 23.5,120.12 23.5,118.17 ARDUINO_NANO1.9 | U2.5 11.75,141.75 v12.75,140.75
  Top 0.61: 20.12,121.75 20.12,121.88 19.5,122.5 19.5,136.88 20.12,137.5
  Bottom 0.5: v20.62,141.12 13,141 v12.75,140.75
SDA  (via drill 0.8)
  Top 0.5: U3.4 20.95,143 v19.88,143 18.62,141.75 18.62,121.5 20.61,119.51 ARDUINO_NANO1.8 | U2.4 10.8,142.8 v10,142
  Bottom 0.5: v10,142 18.88,142 v19.88,143

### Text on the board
tPlace: TRIG | A | C | RADIOSCH.EU
bPlace: RADIOSCH.EU | N | L | COM | +5V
